VAR_GLOBAL
	AxisArray					               : ARRAY [1..7] OF Axis_REF;//轴变量：包括机械臂、旋转轴和笛卡尔坐标系轴	
    stGroupRef			                       : AXES_GROUP_REF;//PickAndPlace中的轴组变量
	{attribute 'TcInitSymbol'}oidConveryorbelt :MC_COORD_REF;//皮带跟随用的变量
	{attribute 'TcInitSymbol'}oidEndNode_Pallet:MC_COORD_REF;//备用
	BeltAxis                                   : Axis_Ref;//皮带
	PickOrPlace                          AT %Q*: BOOL; //气阀开合
	MaterialNum                                : INT;  //物料个数
	CutterNum                                  : INT;  //物料个数，对比用
	MasterCutterRef                   	       : LREAL; //记录皮带当前位置
	Cutter_Master,Cutter_Slave        	       : Axis_Ref; //旋切主从轴
	gfbPushPopCutter1,gfbPushPopCutter2        : FB_PushPopCutter;	 //队列功能块
	gArrayCutterEnc1,gArrayCutterEnc2		   : ARRAY[1..inum]OF LREAL; //队列数组
	gbPushPopCutterBusy1,gbPushPopCutterBusy2  : BOOL; //队列标志位
	gCurrentMaterial					       : DUT_material; //物料数据结构体
	gCurrentCutterEnc1,gCurrentCutterEnc2      : LREAL; //队列变量
	gCurrentCutterEncNull1,gCurrentCutterEncNull2 :	LREAL; //空队列，用于比较
    stKinToPlc	AT %I*		                      : NcToPlc_NciChannel_Ref;//机器人变量
	stPlcToKin	AT %Q*		                      : PLCTONC_NCICHANNEL_REF;//机器人变量
	AllowToPlace                                  : BOOL  := TRUE; // 允许放置物料
END_VAR
